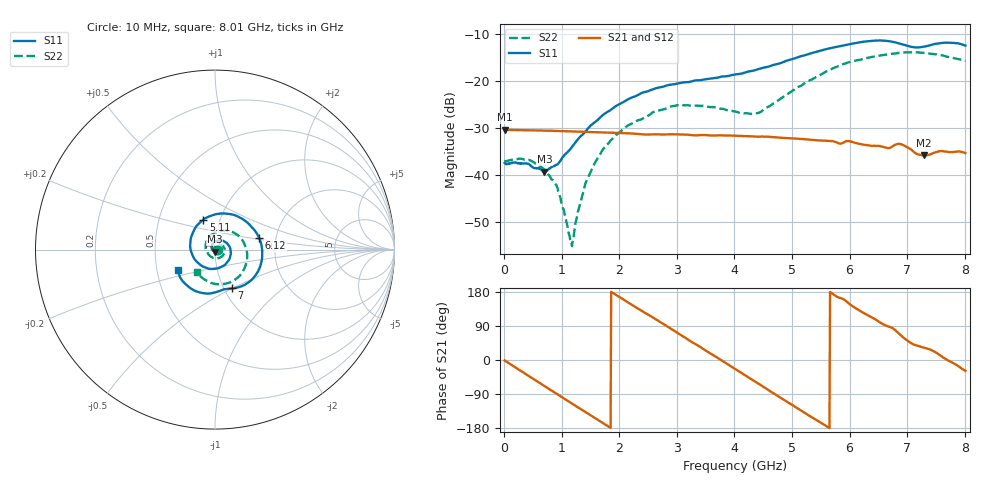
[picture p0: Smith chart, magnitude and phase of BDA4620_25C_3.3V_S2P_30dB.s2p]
!Agilent Technologies,E5071B,MY42404982,A.09.10
!Date: Wed May 06 08:55:23 2026
!Data & Calibration Information:
!Freq	S11:SOLT2(ON)	S21:SOLT2(ON)	S12:SOLT2(ON)	S22:SOLT2(ON)
# Hz S RI R 50
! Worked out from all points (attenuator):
!   801 points, 10 MHz to 8.01 GHz, reference 50 ohm
!   highest |S21| = -30.36 dB at 20 MHz (marker M1); lowest = -35.8 dB at 7.29 GHz (marker M2)
!   lowest |S11| = -39.3 dB at 700 MHz (marker M3), VSWR 1.02, Z = 49.8 - j1.06 ohm
!   |S11| at or under -10 dB: start of sweep to end of sweep
!   |S22| runs from -55.1 to -13.9 dB; largest |S21 - S12| = 0.00015
!   S11 on the Smith chart (normalised r, x): 10 MHz: 1.03, -0.00; 5.11 GHz: 0.83, +0.29; 6.12 GHz: 1.63, +0.23; 7 GHz: 1.09, -0.50; 8.01 GHz: 0.64, -0.15
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1e7  0.0134 -0.000813  0.0303 -0.000637  0.0304 -0.000624  0.014 -0.000432
2e7  0.0132 -0.00087  0.0303 -0.0011  0.0304 -0.0012  0.0141 -0.000347
4.4e8  0.00803 -0.0102  0.0218 -0.0205  0.0218 -0.0205  0.0135 -0.00509
7e8  -0.00186 -0.0107  0.0109 -0.0276  0.0109 -0.0276  0.00905 -0.00707
9.3e8  -0.0118 -0.00548  -0.000425 -0.0294  -0.000416 -0.0294  0.00364 -0.00628
1.16e9  -0.0182 0.0062  -0.0114 -0.0268  -0.0114 -0.0268  -0.00148 -0.0012
1.2e9  -0.0188 0.00874  -0.0131 -0.0259  -0.0131 -0.0259  -0.00206 -1.94e-05
1.35e9  -0.0188 0.0187  -0.019 -0.0217  -0.0191 -0.0217  -0.0036 0.00449
1.53e9  -0.0141 0.0316  -0.0244 -0.015  -0.0244 -0.015  -0.00338 0.0112
1.77e9  0.000671 0.0458  -0.028 -0.00423  -0.028 -0.00423  0.000639 0.0204
2.15e9  0.0383 0.0508  -0.0246 0.013  -0.0246 0.0131  0.0169 0.0291
2.68e9  0.0846 0.00777  -0.00612 0.0264  -0.00605 0.0264  0.0442 0.0196
3.08e9  0.0805 -0.052  0.0114 0.0244  0.0115 0.0244  0.0551 -0.00706
4.01e9  -0.0744 -0.0904  0.0241 -0.0104  0.0241 -0.0105  -0.0101 -0.0463
4.43e9  -0.1341 -0.00763  0.0114 -0.0229  0.0115 -0.0229  -0.0444 -0.0118
5.11e9  -0.0651 0.1671  -0.0152 -0.0189  -0.0154 -0.0189  -0.0168 0.0848
5.35e9  0.00896 0.1981  -0.0208 -0.0113  -0.0208 -0.0113  0.0229 0.1015
6.12e9  0.2452 0.0657  -0.0155 0.0154  -0.0155 0.0154  0.161 0.038
6.68e9  0.204 -0.1684  0.000719 0.0193  0.000717 0.0194  0.1701 -0.09
7e9  0.0951 -0.216  0.0123 0.0154  0.0123 0.0155  0.1238 -0.1579
7.29e9  0.0278 -0.2295  0.0136 0.00871  0.0137 0.00881  0.0554 -0.1907
8.01e9  -0.2083 -0.1138  0.015 -0.00817  0.0151 -0.0082  -0.1013 -0.1276
